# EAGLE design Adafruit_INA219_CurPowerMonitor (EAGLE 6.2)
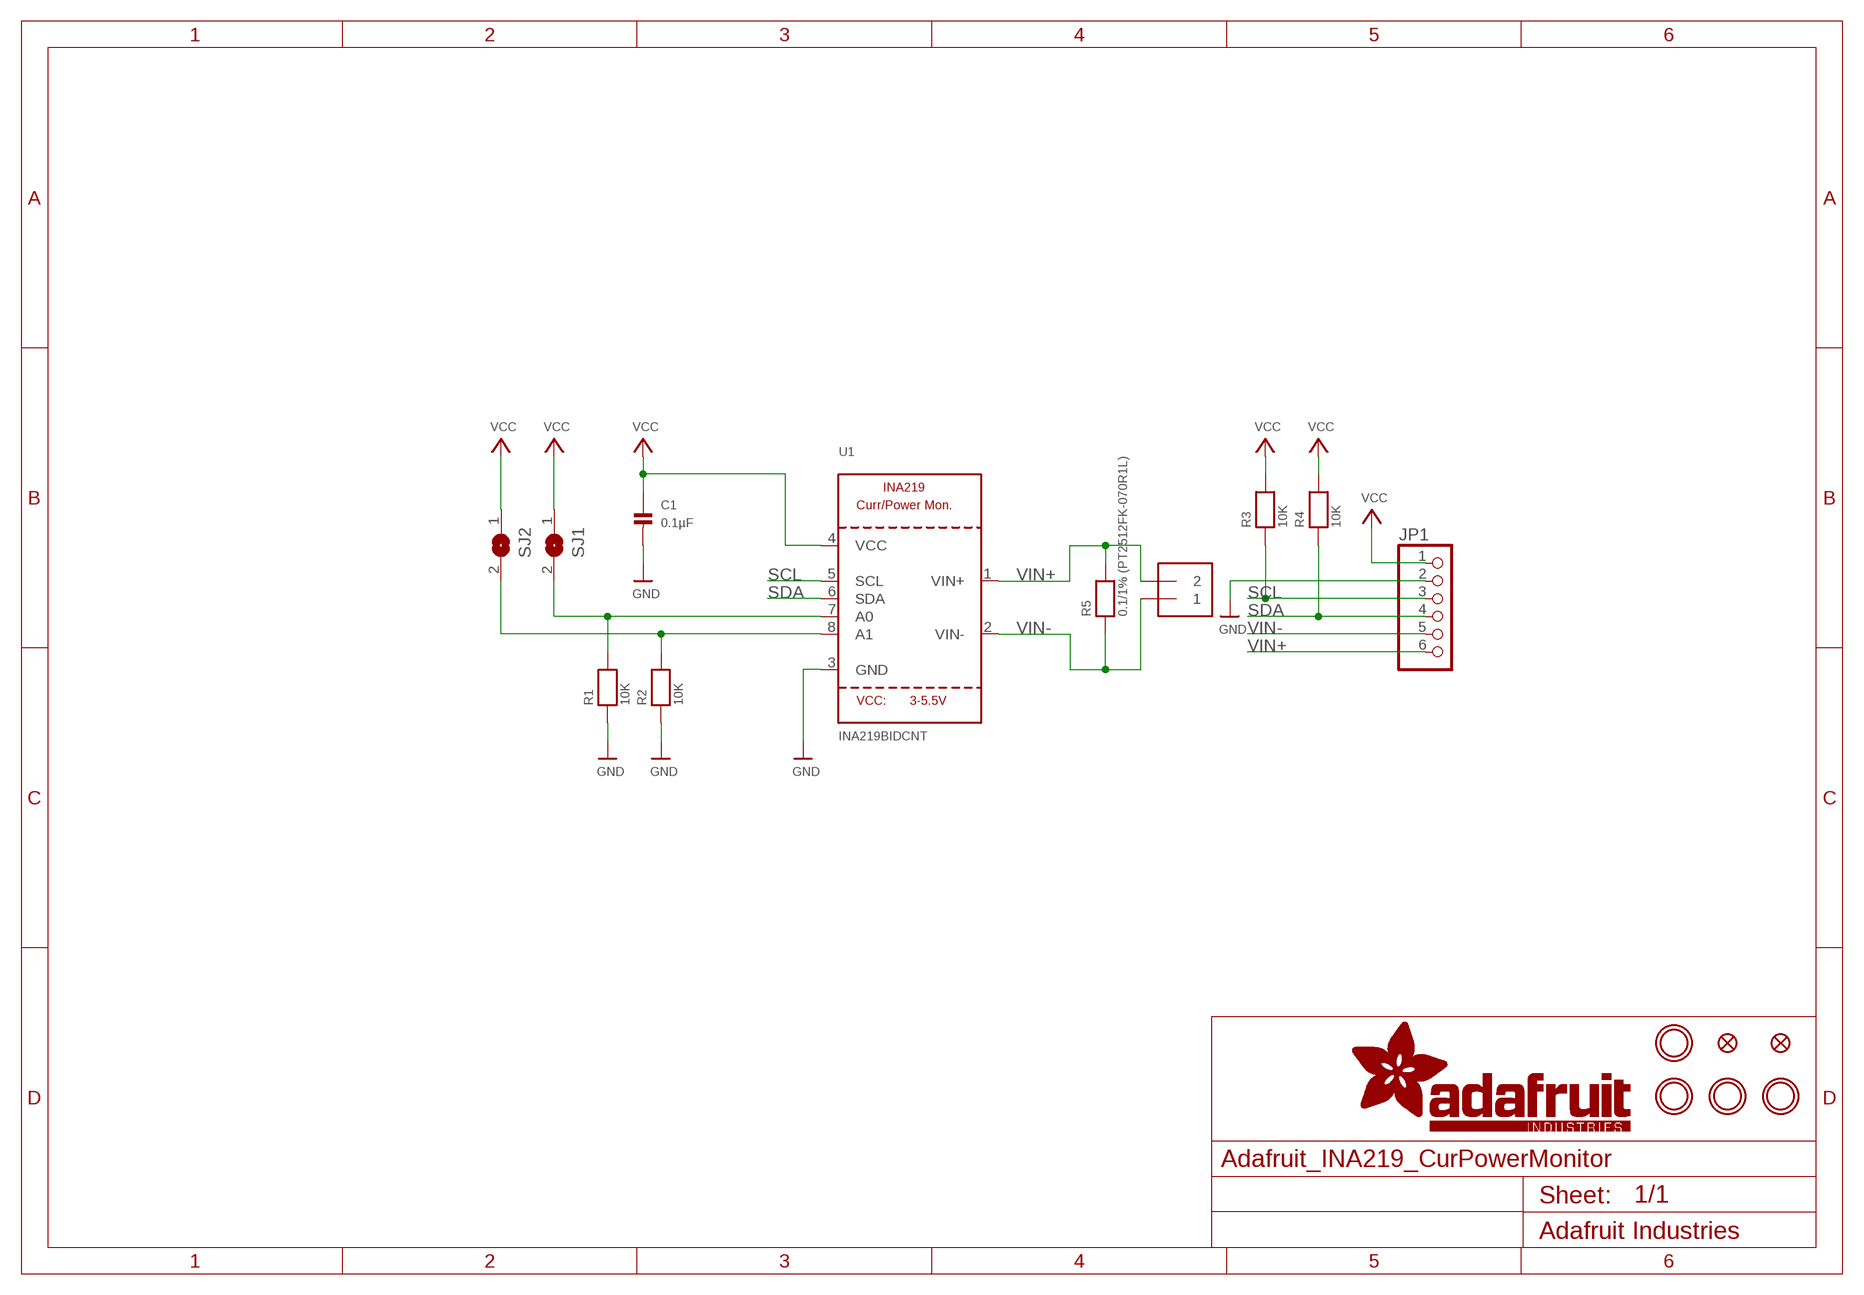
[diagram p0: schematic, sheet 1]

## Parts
C1  0.1µF  CAP_CERAMIC0805  [0805]
FID1  FIDUCIAL""  [FIDUCIAL_1MM]
FID2  FIDUCIAL""  [FIDUCIAL_1MM]
J1  TERMBLOCK_1X2-3.5MM  [1X2-3.5MM]
JP1  HEADER-1X670MIL  [1X06_ROUND_70]
R1  10K  RESISTOR0805  [0805]
R2  10K  RESISTOR0805  [0805]
R3  10K  RESISTOR0805  [0805]
R4  10K  RESISTOR0805  [0805]
R5  0.1/1% (PT2512FK-070R1L)  RESISTOR2512  [2512]
SJ1  SOLDERJUMPERREFLOW_NOPASTE  [SOLDERJUMPER_REFLOW_NOPASTE]
SJ2  SOLDERJUMPERREFLOW_NOPASTE  [SOLDERJUMPER_REFLOW_NOPASTE]
U1  INA219BIDCNT  INA219  [SOT23-8]
U$7  MOUNTINGHOLE2.5  [MOUNTINGHOLE_2.5_PLATED]
U$8  MOUNTINGHOLE2.5  [MOUNTINGHOLE_2.5_PLATED]
U$9  MOUNTINGHOLE2.5  [MOUNTINGHOLE_2.5_PLATED]
U$10  MOUNTINGHOLE2.5  [MOUNTINGHOLE_2.5_PLATED]

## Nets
GND: C1.2 JP1.2 R1.1 R2.1 U1.3(GND)
N$1: R2.2 SJ2.2 U1.8(A1)
N$2: R1.2 SJ1.2 U1.7(A0)
SCL: JP1.3 R3.1 U1.5(SCL)
SDA: JP1.4 R4.1 U1.6(SDA)
VCC: C1.1 JP1.1 R3.2 R4.2 SJ1.1 SJ2.1 U1.4(VCC)
VIN+: J1.2 JP1.6 R5.2 U1.1(VIN+)
VIN-: J1.1 JP1.5 R5.1 U1.2(VIN-)

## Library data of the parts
C1 = microbuilder:CAP_CERAMIC: Ceramic Capacitors
FID1 FID2 = microbuilder:FIDUCIAL: Fiducial Alignment Points
J1 = microbuilder:TERMBLOCK_1X2: 3.5mm Terminal block
JP1 = microbuilder:HEADER-1X6: PIN HEADER
R1-R5 = microbuilder:RESISTOR: Resistors
SJ1 SJ2 = microbuilder:SOLDERJUMPER: SMD Solder JUMPER
U1 = microbuilder:INA219: INA219 - I2C Current/Power Monitor Voltage Range: 0-26V Accuracy: 0.5% Temperature: -40°C - 125°C
U$7-U$10 = microbuilder:MOUNTINGHOLE: Mounting Hole

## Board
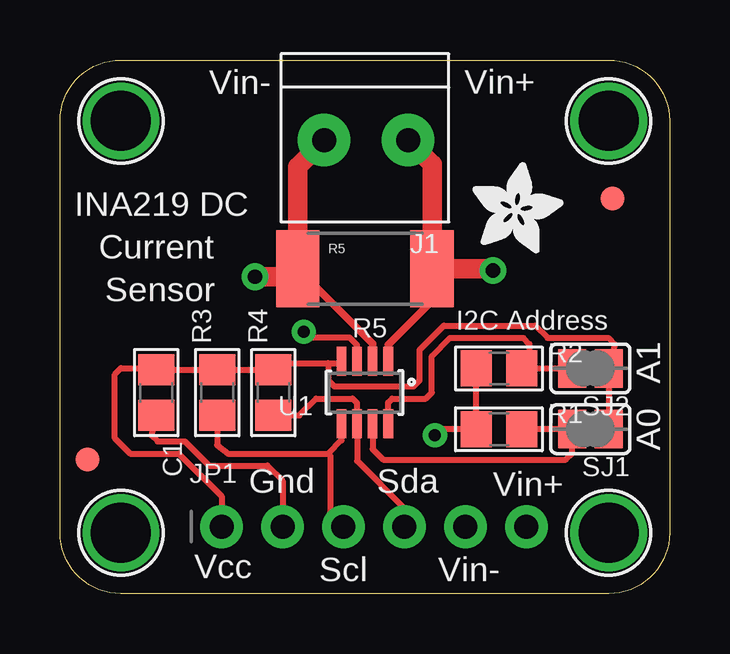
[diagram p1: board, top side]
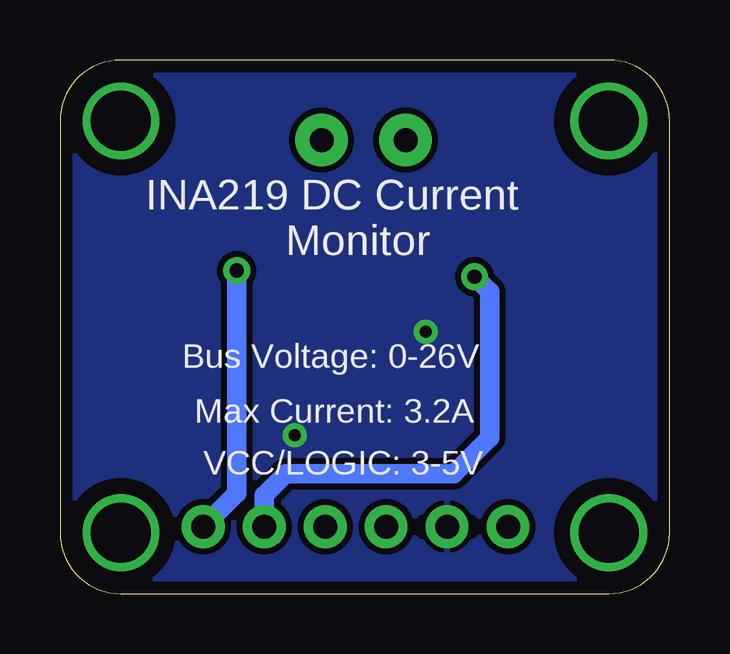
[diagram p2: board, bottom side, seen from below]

Size 25.4 x 22.24 mm. Coordinates in mm from the lower left corner, seen from the top.
Outline: 0,2.54 0,19.7 arc-90 2.54,22.24 22.86,22.24 arc-90 25.4,19.7 25.4,2.54 arc-90 22.86,0 2.54,0 arc-90 0,2.54
Copper layers (1*16): Top 0.035mm / dielectric 1.5mm / Bottom 0.035mm
Design rules: minimum track width 8mil, minimum drill 0.4mm, track to track 8mil, track to pad 8mil, pad to pad 8mil, via to via 8mil, smd to smd 8mil, copper to edge 20mil, drill to drill 8mil, minimum pad ring 8mil, minimum via ring 10mil, stop-mask expansion 3mil, vias tented up to drill 0mil, thermal gap 8mil
bRestrict: area 10.2,2.5 to 10.3,3; area 8.3,2.5 to 8.4,3

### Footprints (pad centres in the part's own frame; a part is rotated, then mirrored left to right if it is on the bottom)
0805 = smd 1.3 x 1.5: 1 -0.95,0; 2 0.95,0
FIDUCIAL_1MM = smd 1 x 1: 1 0,0
1X2-3.5MM = drill 1 pad 2.184: 1 1.8,0; 2 -1.7,0
1X06_ROUND_70 = drill 1 pad 1.778: 1 -6.35,0; 2 -3.81,0; 3 -1.27,0; 4 1.27,0; 5 3.81,0; 6 6.35,0
2512 = smd 1.8 x 3.2: 1 -2.8,0; 2 2.8,0
SOLDERJUMPER_REFLOW_NOPASTE = smd 1.168 x 1.6: 1 -0.762,0; 2 0.762,0
SOT23-8 = smd 0.4 x 1.2: 1 -0.975,-1.3; 2 -0.325,-1.3; 3 0.325,-1.3; 4 0.975,-1.3; 5 0.975,1.3; 6 0.325,1.3; 7 -0.325,1.3; 8 -0.975,1.3
MOUNTINGHOLE_2.5_PLATED = drill 2.5 pad 3.2: P$1 0,0

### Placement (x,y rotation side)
C1  4.01,8.38 270 top
FID1  23.01,16.46 0 top
FID2  1.14,5.59 0 top
J1  12.8,18.9 180 top
JP1  13.08,2.79 0 top
R1  18.29,6.86 0 top
R2  18.29,9.39 0 top
R3  6.55,8.38 90 top
R4  8.89,8.38 90 top
R5  12.7,13.54 0 top
SJ1  22.1,6.86 180 top
SJ2  22.1,9.39 180 top
U1  12.7,8.38 180 top
U$7  22.86,2.54 0 top
U$8  2.54,2.54 0 top
U$9  2.54,19.7 0 top
U$10  22.86,19.7 0 top
U$11  [ADAFRUIT_3.5MM]  17.17,14.18 0 top

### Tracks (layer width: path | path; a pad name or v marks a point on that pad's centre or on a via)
GND  (via drill 0.5)
  Top 0.254: R2.1 R1.1 15.88,6.86 v15.62,6.6 | U1.3 12.38,10.36 12.06,10.67 10.41,10.67 v10.16,10.92 | C1.2 3.81,6.6 4.06,6.35 5.21,6.35 6.22,5.33 8.64,5.33 9.27,4.7 JP1.2 9.14,2.92
  Bottom 0.254: v15.62,6.6 15.62,6.48 | v10.16,10.92 9.91,10.92
  pour Bottom (isolate 0.254): 0,0 0,22.24 26.67,22.24 26.67,0
N$1
  Top 0.254: SJ2.2 R2.2 19.56,9.46 19.56,10.41 19.3,10.66 16.25,10.66 15.49,9.91 15.49,8.38 15.24,8.13 13.84,8.13 13.68,7.96 U1.8
N$2
  Top 0.254: R1.2 SJ1.2 21.34,5.84 21.08,5.59 13.46,5.59 13.03,6.03 U1.7
SCL
  Top 0.254: R3.1 6.55,6.2 7,5.84 11.18,5.84 | 11.18,5.84 11.25,5.77 11.25,3.35 JP1.3 | U1.5 11.72,6.39 11.18,5.84
SDA
  Top 0.254: R4.1 9.97,7.43 10.67,8.13 12.19,8.13 12.38,7.95 U1.6 12.38,5.53 14.35,3.56 JP1.4
VCC
  Top 0.254: SJ1.1 SJ2.1 23.11,10.41 22.86,10.66 20.32,10.66 19.81,11.17 15.99,11.17 14.99,10.16 14.99,8.89 14.73,8.64 11.43,8.64 11.18,8.89 11.18,9.61 | 11.18,9.61 9.17,9.61 R4.2 R3.2 C1.1 3.74,9.4 2.54,9.4 2.29,9.14 2.29,6.48 2.92,5.84 4.95,5.84 6.73,4.06 JP1.1 | 11.18,9.61 11.65,9.61 U1.4
VIN+  (via drill 0.6)
  Top 0.305: U1.1 13.68,10.37 15.49,12.19 R5.2
  Top 0.813: J1.2 15.5,17.9 R5.2 17.95,13.54 v18.03,13.46
  Bottom 0.813: JP1.6 18.03,4.19 v18.03,13.46
VIN-  (via drill 0.6)
  Top 0.305: U1.2 13.03,10.42 R5.1
  Top 0.813: v8.13,13.21 9.57,13.21 R5.1 9.9,17.8 J1.1
  Bottom 0.813: JP1.5 16.89,4.11 16,5 9,5 7.5,6.5 7.5,12.58 v8.13,13.21

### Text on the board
tPlace: Vin- | Vin+ | INA219 DC | Current | Sensor | R5 | I2C Address | A1 | A0 | Gnd | Sda | Vin+ | Vcc | Scl | Vin-
bPlace: INA219 DC Current | Monitor | Bus Voltage: 0-26V | Max Current: 3.2A | VCC/LOGIC: 3-5V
